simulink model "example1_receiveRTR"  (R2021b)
settings: Solver=FixedStepDiscrete  StartTime=0.0  StopTime=inf  FixedStep=0.2  RelTol=1e-3
libraries: CANBusLib x3

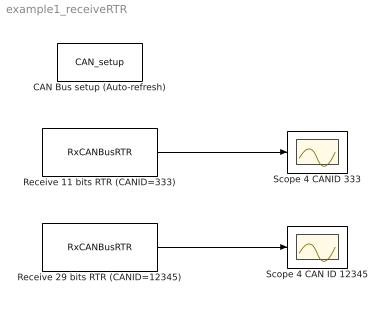
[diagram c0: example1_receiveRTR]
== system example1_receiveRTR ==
  CAN Bus setup (Auto-refresh) : CANBusLib/CAN_setup  Priority=1  g1_cmbPortName="\"COM17\""  g2_cmbBaudRate=250000  g3_chkEcho=off  g59_chkTerminator=on  g4_cmbObjectID=0  g5_chkEnableSync=off  g10_chkRxWDEnable=off  g12_cmbRxWDLen=1  g13_cmbRxWDStartPos=1  g_60_cmbRxWDMode=0  g15_chkTxWDEnable=off  g17_cmbTxWDLen=1  g18_cmbTxWDStartPos=1  g_61_cmbTxWDMode=0  g20_ediF1=0  g21_chkExt4F1=off  g22_ediF2=0  g23_chkExt4F2=off  g24_ediF3=0  g25_chkExt4F3=off  g26_ediF4=0  g27_chkExt4F4=off  g28_ediF5=0  g29_chkExt4F5=off  g30_ediF6=0  g31_chkExt4F6=off  g32_ediF7=0  g33_chkExt4F7=off  g34_ediF8=0  g35_chkExt4F8=off  g36_ediM1=0  g37_ediF9=0  g38_chkExt4F9=on  g39_ediF10=0  g40_chkExt4F10=on  g41_ediF11=0  g42_chkExt4F11=on  g43_ediF12=0  g44_chkExt4F12=on  g45_ediM2=0  g46_ediF13=0  g47_chkExt4F13=off  g48_ediF14=0  g49_chkExt4F14=on  g50_ediF15=0  g51_chkExt4F15=on  g52_ediF16=0  g53_chkExt4F16=on  g54_ediM3=0  g62_autoFresh=on
  Receive 11 bits RTR (CANID=333) : CANBusLib/RxCANBusRTR  g1_ObjectID=0  g2_CANID=0  g3_Extended=off
  Receive 29 bits RTR (CANID=12345) : CANBusLib/RxCANBusRTR  g1_ObjectID=0  g2_CANID=0  g3_Extended=off
  Scope 4 CAN ID 12345 : Scope
  Scope 4 CANID 333 : Scope
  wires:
  Receive 11 bits RTR (CANID=333)/1 -> Scope 4 CANID 333/1
  Receive 29 bits RTR (CANID=12345)/1 -> Scope 4 CAN ID 12345/1
